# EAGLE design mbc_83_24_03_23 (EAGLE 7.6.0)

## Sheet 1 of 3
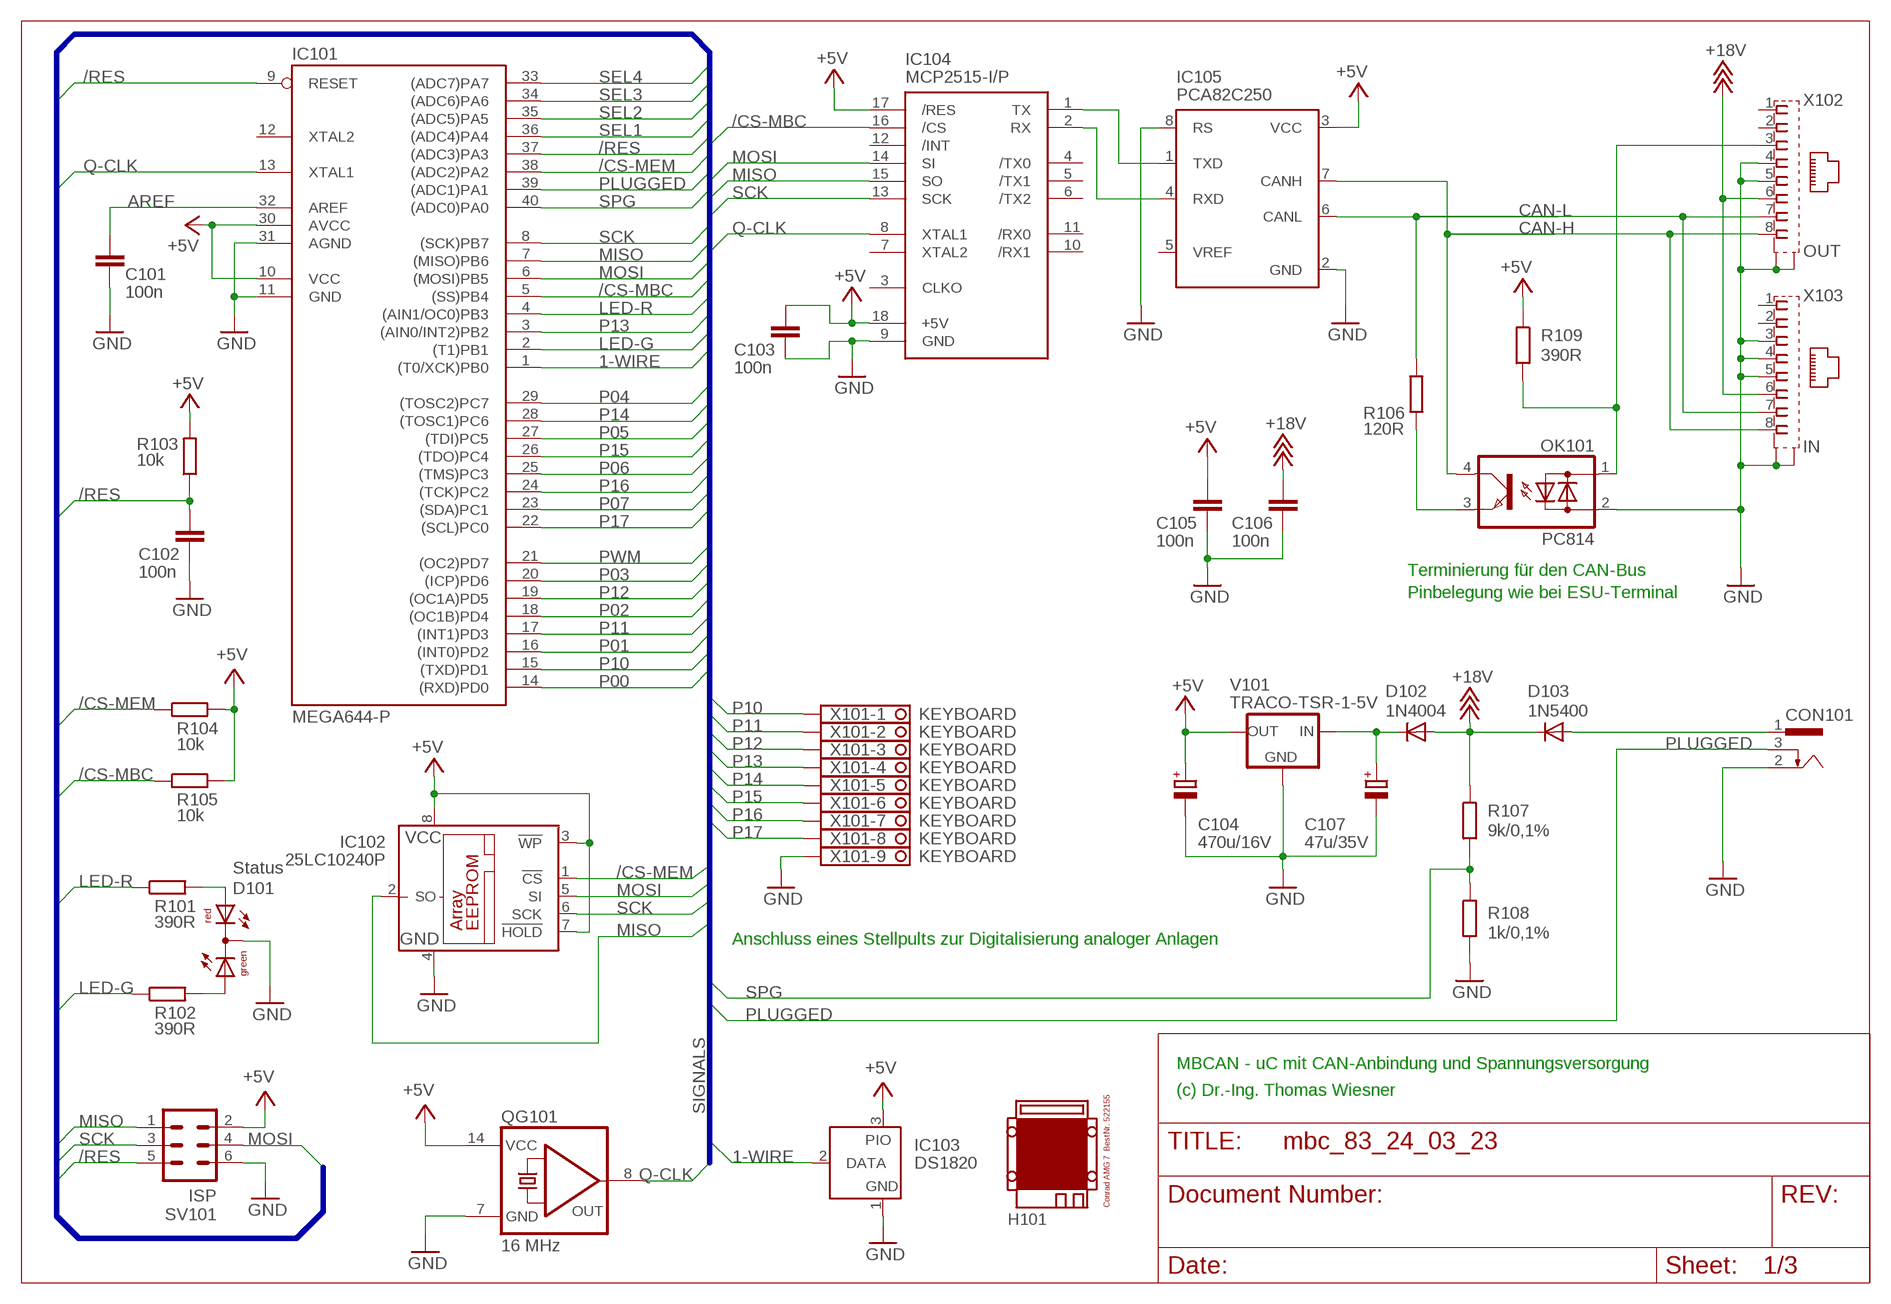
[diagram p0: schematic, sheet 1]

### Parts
C101  100n  C-EU025-025X050  [C025-025X050]
C102  100n  C-EU025-025X050  [C025-025X050]
C103  100n  C-EU025-025X050  [C025-025X050]
C104  470u/16V  CPOL-EUE3.5-8  [E3,5-8]
C105  100n  C-EU025-025X050  [C025-025X050]
C106  100n  C-EU025-025X050  [C025-025X050]
C107  47u/35V  CPOL-EUE2.5-7  [E2,5-7]
CON101  POWER-JACK  [POWER-JACK]
D101  Status  DUOLED5MM  [DUOLED5MM]
D102  1N4004  [DO41-10]
D103  1N5400  [DO201-15]
H101  MODULGEHÄUSE-AMG-7  [MODULGEHÄUSE-AMG-7]
IC101  MEGA644-P  MEGA323-P  [DIL40]
IC102  25LC10240P  25LC040P  [DIL8]
IC103  DS1820  DS2405  [TO92-]
IC104  MCP2515-I/P  MCP2510-I/P  [DIL18]
IC105  PCA82C250  [DIL08]
OK101  PC814  [DIL04]
QG101  16 MHz  QG5860  [DIL14S]
R101  390R  R-EU_0207/10  [0207/10]
R102  390R  R-EU_0207/10  [0207/10]
R103  10k  R-EU_0207/10  [0207/10]
R104  10k  R-EU_0207/10  [0207/10]
R105  10k  R-EU_0207/10  [0207/10]
R106  120R  R-EU_0207/10  [0207/10]
R107  9k/0,1%  R-EU_0207/10  [0207/10]
R108  1k/0,1%  R-EU_0207/10  [0207/10]
R109  390R  R-EU_0207/10  [0207/10]
SV101  ISP  ML6  [ML6]
V101  TRACO-TSR-1-5V  [TRACO-TSR-1]
X101  KEYBOARD  1751316  [1751316]
X102  OUT  0446200002  [0446200002]
X103  IN  0446200002  [0446200002]

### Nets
1-WIRE: IC101.1((T0/XCK)PB0) IC103.2(DATA)
+5V: C103.1 C104.+ C105.1 IC101.10(VCC) IC101.30(AVCC) IC102.3(!WP) IC102.7(!HOLD) IC102.8(VCC) IC103.3(PIO) IC104.17(/RES) IC104.18(+5V) IC105.3(VCC) QG101.14(VCC) R103.2 R104.2 R105.2 R109.1 SV101.2 V101.OUT ; also sheet 2
+18V: C106.1 D102.A D103.C R107.1 X102.6 X103.6 ; also sheet 2,3
/CS-MBC: IC101.5((SS)PB4) IC104.16(/CS) R105.1
/CS-MEM: IC101.38((ADC2)PA2) IC102.1(!CS) R104.1
/RES: C102.1 IC101.9(RESET) IC101.37((ADC3)PA3) R103.1 SV101.5
AREF: C101.1 IC101.32(AREF)
CAN-H: IC105.7(CANH) OK101.4(C) X102.8 X103.8
CAN-L: IC105.6(CANL) R106.2 X102.7 X103.7
GND: C101.2 C102.2 C103.2 C104.- C105.2 C106.2 C107.- CON101.2 D101.K(C) IC101.11(GND) IC101.31(AGND) IC102.4(GND) IC103.1(GND) IC104.9(GND) IC105.2(GND) IC105.8(RS) OK101.2(AC2) QG101.7(GND) R108.2 SV101.6 V101.GND X101.9 X102.4 X102.5 X102.S@1(S1) X102.S@2(S2) X103.3 X103.4 X103.5 X103.S@1(S1) X103.S@2(S2) ; also sheet 2,3
LED-G: IC101.2((T1)PB1) R102.1
LED-R: IC101.4((AIN1/OC0)PB3) R101.1
MISO: IC101.7((MISO)PB6) IC102.2(SO) IC104.15(SO) SV101.1
MOSI: IC101.6((MOSI)PB5) IC102.5(SI) IC104.14(SI) SV101.4
N$1: IC104.1(TX) IC105.1(TXD)
N$2: IC104.2(RX) IC105.4(RXD)
N$3: OK101.3(E) R106.1
N$5: OK101.1(AC1) R109.2 X102.3
N$6: C107.+ D102.C V101.IN
N$9: D101.AR R101.2
N$13: D101.AG R102.2
P00: IC101.14((RXD)PD0) ; also sheet 2
P01: IC101.16((INT0)PD2) ; also sheet 2
P02: IC101.18((OC1B)PD4) ; also sheet 2
P03: IC101.20((ICP)PD6) ; also sheet 2
P04: IC101.29((TOSC2)PC7) ; also sheet 2
P05: IC101.27((TDI)PC5) ; also sheet 2
P06: IC101.25((TMS)PC3) ; also sheet 2
P07: IC101.23((SDA)PC1) ; also sheet 2
P10: IC101.15((TXD)PD1) X101.1
P11: IC101.17((INT1)PD3) X101.2
P12: IC101.19((OC1A)PD5) X101.3
P13: IC101.3((AIN0/INT2)PB2) X101.4
P14: IC101.28((TOSC1)PC6) X101.5
P15: IC101.26((TDO)PC4) X101.6
P16: IC101.24((TCK)PC2) X101.7
P17: IC101.22((SCL)PC0) X101.8
PLUGGED: CON101.3 IC101.39((ADC1)PA1)
PWM: IC101.21((OC2)PD7) ; also sheet 3
Q-CLK: IC101.13(XTAL1) IC104.8(XTAL1) QG101.8(OUT)
SCK: IC101.8((SCK)PB7) IC102.6(SCK) IC104.13(SCK) SV101.3
SEL1: IC101.36((ADC4)PA4) ; also sheet 2
SEL2: IC101.35((ADC5)PA5) ; also sheet 2
SEL3: IC101.34((ADC6)PA6) ; also sheet 2
SEL4: IC101.33((ADC7)PA7) ; also sheet 2
SPG: IC101.40((ADC0)PA0) R107.2 R108.1
V-NETZTEIL1: CON101.1 D103.A
Unconnected: IC101.12(XTAL2) IC104.3(CLKO) IC104.4(/TX0) IC104.5(/TX1) IC104.6(/TX2) IC104.7(XTAL2) IC104.10(/RX1) IC104.11(/RX0) IC104.12(/INT) IC105.5(VREF) X102.1 X102.2 X103.1 X103.2

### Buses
SIGNALS

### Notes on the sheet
- Terminierung für den CAN-Bus
- Pinbelegung wie bei ESU-Terminal
- Anschluss eines Stellpults zur Digitalisierung analoger Anlagen
- MBCAN - uC mit CAN-Anbindung und Spannungsversorgung
- (c) Dr.-Ing. Thomas Wiesner

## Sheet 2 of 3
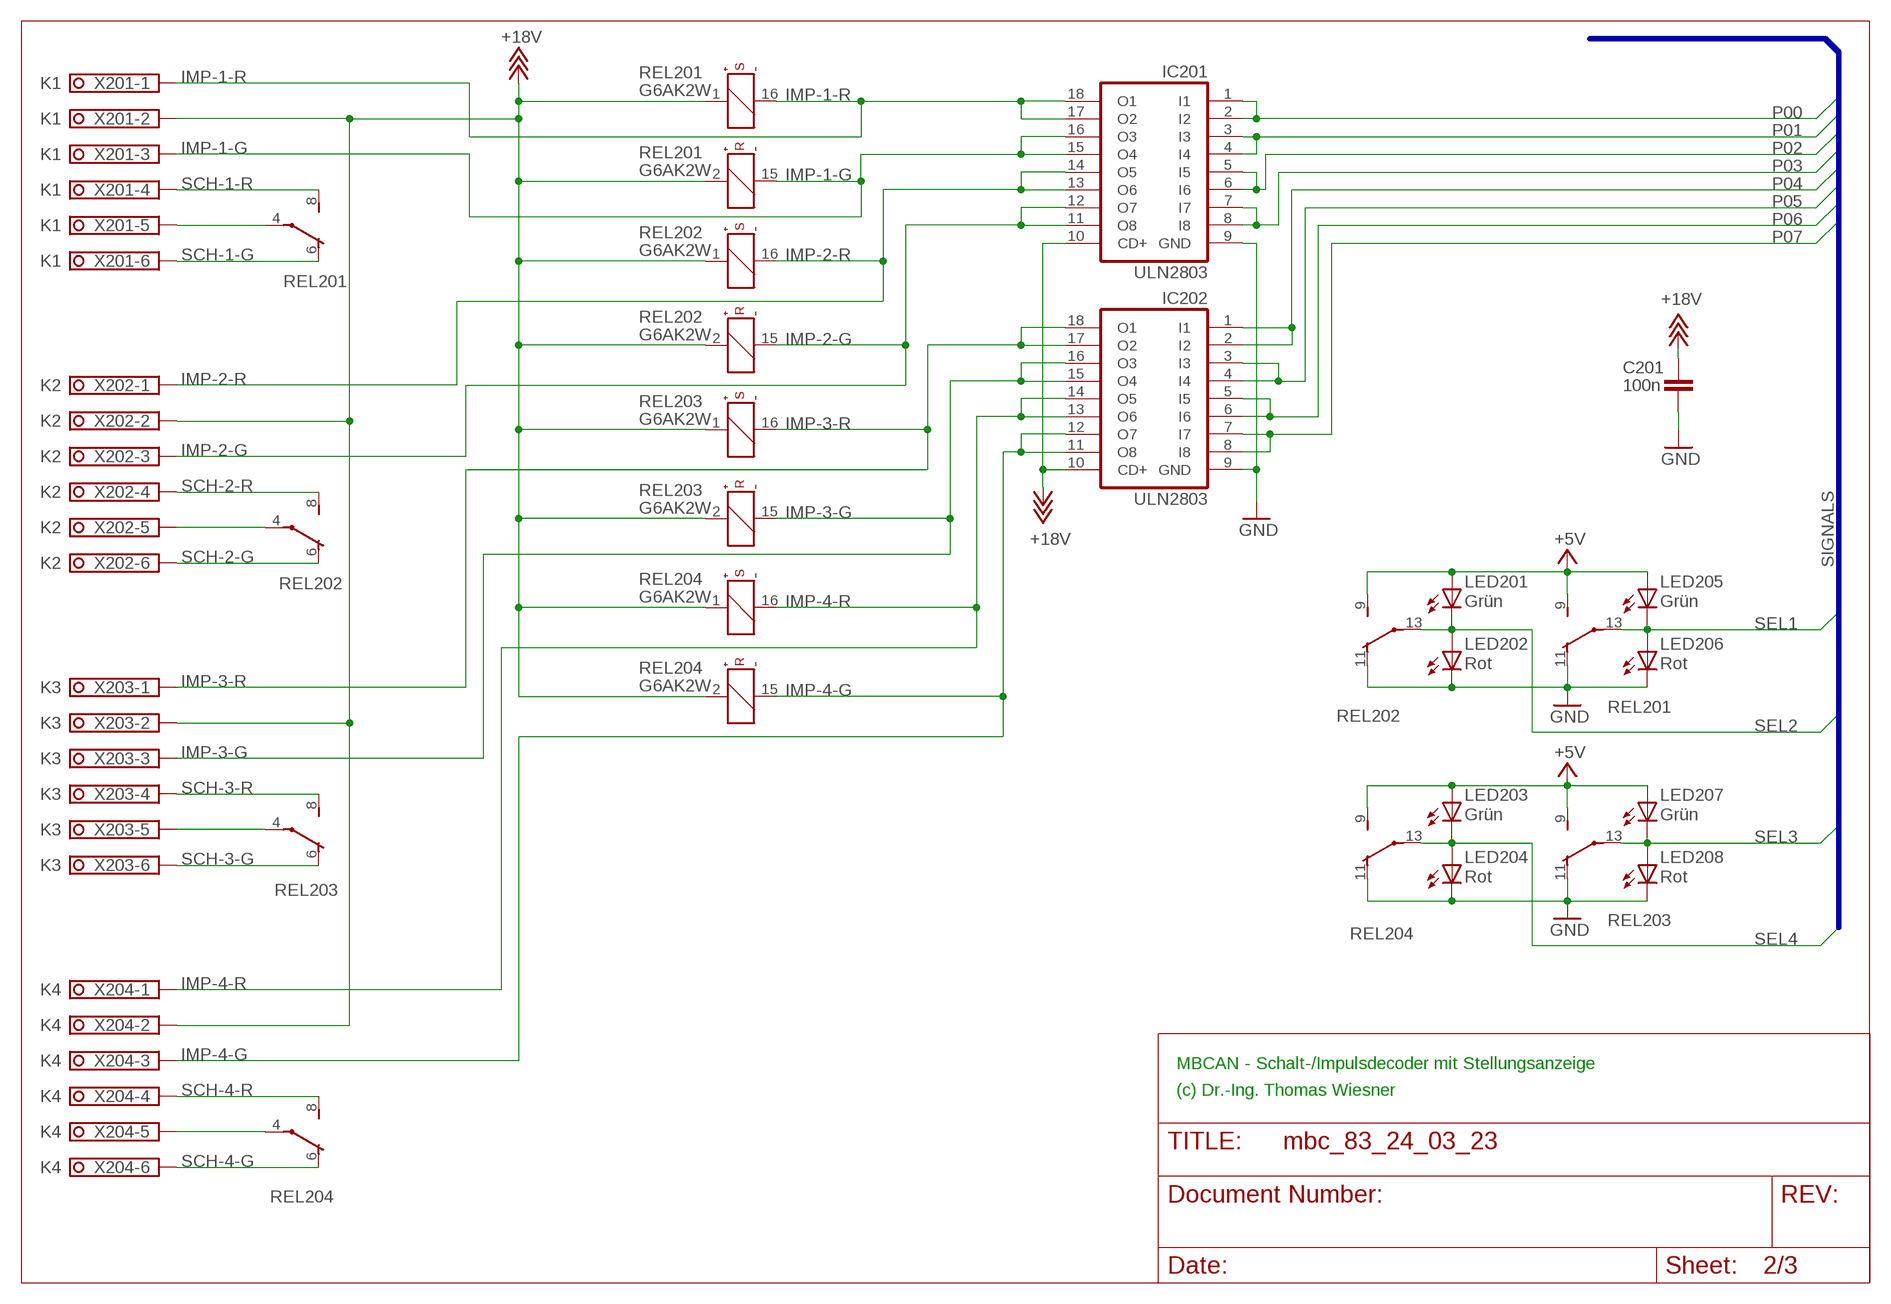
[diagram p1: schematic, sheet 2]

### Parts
C201  100n  C-EU025-025X050  [C025-025X050]
IC201  ULN2803  ULN2803A  [DIL18]
IC202  ULN2803  ULN2803A  [DIL18]
LED201  Grün  LED3MM  [LED3MM]
LED202  Rot  LED3MM  [LED3MM]
LED203  Grün  LED3MM  [LED3MM]
LED204  Rot  LED3MM  [LED3MM]
LED205  Grün  LED3MM  [LED3MM]
LED206  Rot  LED3MM  [LED3MM]
LED207  Grün  LED3MM  [LED3MM]
LED208  Rot  LED3MM  [LED3MM]
REL201  G6AK2W  [REL-BIPOLAR]
REL202  G6AK2W  [REL-BIPOLAR]
REL203  G6AK2W  [REL-BIPOLAR]
REL204  G6AK2W  [REL-BIPOLAR]
X201  K1  1751280  [1751280]
X202  K2  1751280  [1751280]
X203  K3  1751280  [1751280]
X204  K4  1751280  [1751280]

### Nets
+5V: LED201.A LED203.A LED205.A LED207.A REL201.9(S) REL202.9(S) REL203.9(S) REL204.9(S) ; also sheet 1
+18V: C201.1 IC201.10(CD+) IC202.10(CD+) REL201.1(+) REL201.2(+) REL202.1(+) REL202.2(+) REL203.1(+) REL203.2(+) REL204.1(+) REL204.2(+) X201.2 X202.2 X203.2 X204.2 ; also sheet 1,3
GND: C201.2 IC201.9(GND) IC202.9(GND) LED202.K(C) LED204.K(C) LED206.K(C) LED208.K(C) REL201.11(O) REL202.11(O) REL203.11(O) REL204.11(O) ; also sheet 1,3
IMP-1-G: IC201.15(O4) IC201.16(O3) REL201.15(-) X201.3 ; also sheet 3
IMP-1-R: IC201.17(O2) IC201.18(O1) REL201.16(-) X201.1 ; also sheet 3
IMP-2-G: IC201.11(O8) IC201.12(O7) REL202.15(-) X202.3 ; also sheet 3
IMP-2-R: IC201.13(O6) IC201.14(O5) REL202.16(-) X202.1 ; also sheet 3
IMP-3-G: IC202.15(O4) IC202.16(O3) REL203.15(-) X203.3 ; also sheet 3
IMP-3-R: IC202.17(O2) IC202.18(O1) REL203.16(-) X203.1 ; also sheet 3
IMP-4-G: IC202.11(O8) IC202.12(O7) REL204.15(-) X204.3 ; also sheet 3
IMP-4-R: IC202.13(O6) IC202.14(O5) REL204.16(-) X204.1 ; also sheet 3
N$12: REL202.4(P) X202.5
N$14: REL201.4(P) X201.5
N$15: REL203.4(P) X203.5
N$16: REL204.4(P) X204.5
P00: IC201.1(I1) IC201.2(I2) ; also sheet 1
P01: IC201.3(I3) IC201.4(I4) ; also sheet 1
P02: IC201.5(I5) IC201.6(I6) ; also sheet 1
P03: IC201.7(I7) IC201.8(I8) ; also sheet 1
P04: IC202.1(I1) IC202.2(I2) ; also sheet 1
P05: IC202.3(I3) IC202.4(I4) ; also sheet 1
P06: IC202.5(I5) IC202.6(I6) ; also sheet 1
P07: IC202.7(I7) IC202.8(I8) ; also sheet 1
SCH-1-G: REL201.6(O) X201.6 ; also sheet 3
SCH-1-R: REL201.8(S) X201.4
SCH-2-G: REL202.6(O) X202.6 ; also sheet 3
SCH-2-R: REL202.8(S) X202.4
SCH-3-G: REL203.6(O) X203.6 ; also sheet 3
SCH-3-R: REL203.8(S) X203.4
SCH-4-G: REL204.6(O) X204.6 ; also sheet 3
SCH-4-R: REL204.8(S) X204.4
SEL1: LED205.K(C) LED206.A REL201.13(P) ; also sheet 1
SEL2: LED201.K(C) LED202.A REL202.13(P) ; also sheet 1
SEL3: LED207.K(C) LED208.A REL203.13(P) ; also sheet 1
SEL4: LED203.K(C) LED204.A REL204.13(P) ; also sheet 1

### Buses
SIGNALS

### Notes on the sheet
- MBCAN - Schalt-/Impulsdecoder mit Stellungsanzeige
- (c) Dr.-Ing. Thomas Wiesner

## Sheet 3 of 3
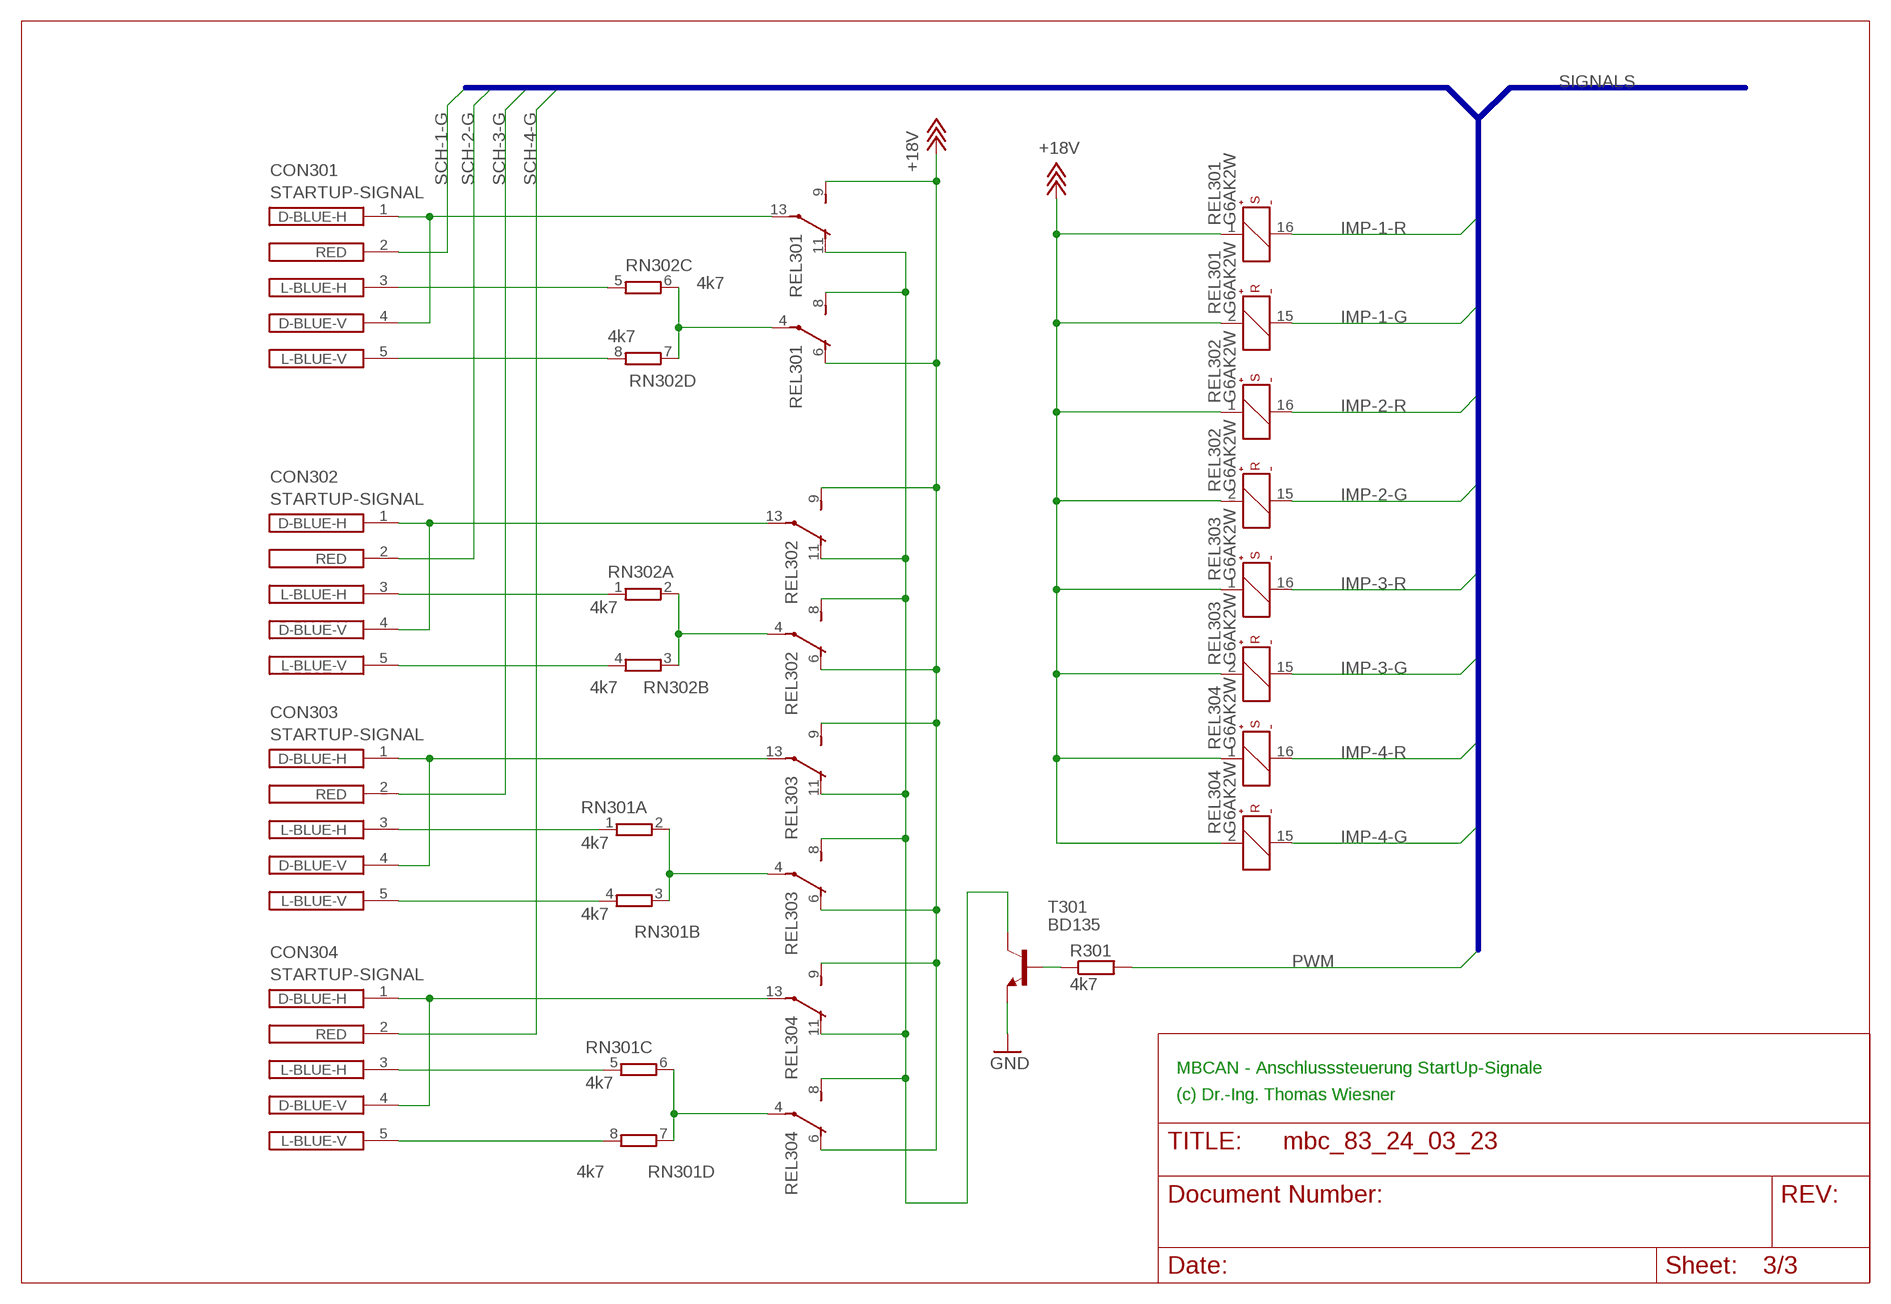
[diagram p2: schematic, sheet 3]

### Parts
CON301  STARTUP-SIGNAL  [SIGNAL-MAIN]
CON302  STARTUP-SIGNAL  [SIGNAL-MAIN]
CON303  STARTUP-SIGNAL  [SIGNAL-MAIN]
CON304  STARTUP-SIGNAL  [SIGNAL-MAIN]
R301  4k7  R-EU_0207/10  [0207/10]
REL301  G6AK2W  [REL-BIPOLAR]
REL302  G6AK2W  [REL-BIPOLAR]
REL303  G6AK2W  [REL-BIPOLAR]
REL304  G6AK2W  [REL-BIPOLAR]
RN301  4k7  E4R  [SIL8]
RN302  4k7  E4R  [SIL8]
T301  BD135  -NPN-TO126V  [TO126V]

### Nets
+18V: REL301.1(+) REL301.2(+) REL301.6(O) REL301.9(S) REL302.1(+) REL302.2(+) REL302.6(O) REL302.9(S) REL303.1(+) REL303.2(+) REL303.6(O) REL303.9(S) REL304.1(+) REL304.2(+) REL304.6(O) REL304.9(S) ; also sheet 1,2
GND: T301.1(E) ; also sheet 1,2
IMP-1-G: REL301.15(-) ; also sheet 2
IMP-1-R: REL301.16(-) ; also sheet 2
IMP-2-G: REL302.15(-) ; also sheet 2
IMP-2-R: REL302.16(-) ; also sheet 2
IMP-3-G: REL303.15(-) ; also sheet 2
IMP-3-R: REL303.16(-) ; also sheet 2
IMP-4-G: REL304.15(-) ; also sheet 2
IMP-4-R: REL304.16(-) ; also sheet 2
N$4: CON302.5(L-BLUE-V) RN302.4
N$7: CON301.1(D-BLUE-H) CON301.4(D-BLUE-V) REL301.13(P)
N$8: CON301.5(L-BLUE-V) RN302.8
N$10: CON303.5(L-BLUE-V) RN301.4
N$11: CON304.5(L-BLUE-V) RN301.8
N$17: R301.1 T301.3(B)
N$18: REL301.8(S) REL301.11(O) REL302.8(S) REL302.11(O) REL303.8(S) REL303.11(O) REL304.8(S) REL304.11(O) T301.2(C)
N$19: CON302.1(D-BLUE-H) CON302.4(D-BLUE-V) REL302.13(P)
N$20: CON302.3(L-BLUE-H) RN302.1
N$21: CON304.1(D-BLUE-H) CON304.4(D-BLUE-V) REL304.13(P)
N$23: CON304.3(L-BLUE-H) RN301.5
N$24: CON303.1(D-BLUE-H) CON303.4(D-BLUE-V) REL303.13(P)
N$26: CON301.3(L-BLUE-H) RN302.5
N$27: CON303.3(L-BLUE-H) RN301.1
N$29: REL301.4(P) RN302.6 RN302.7
N$30: REL302.4(P) RN302.2 RN302.3
N$31: REL303.4(P) RN301.2 RN301.3
N$32: REL304.4(P) RN301.6 RN301.7
PWM: R301.2 ; also sheet 1
SCH-1-G: CON301.2(RED) ; also sheet 2
SCH-2-G: CON302.2(RED) ; also sheet 2
SCH-3-G: CON303.2(RED) ; also sheet 2
SCH-4-G: CON304.2(RED) ; also sheet 2

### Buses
SIGNALS

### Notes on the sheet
- MBCAN - Anschlusssteuerung StartUp-Signale
- (c) Dr.-Ing. Thomas Wiesner

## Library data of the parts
C101-C103 C105 C106 C201 = rcl:C-EU: CAPACITOR, European symbol
C104 C107 = rcl:CPOL-EU: POLARIZED CAPACITOR, European symbol
CON101 = mbc:POWER-JACK: Power-Stecker für 2,5 mm Hohlbuchse
CON301-CON304 = mbc:STARTUP-SIGNAL: Connector für StartUp-Signale
D101 = led:DUOLED5MM: DUO LED 2 colors, 5 mm, round
D102 = diode:1N4004: DIODE
D103 = diode:1N5400: DIODE
H101 = mbc:MODULGEHÄUSE-AMG-7: Gehäuse
IC101 = atmel:MEGA323-P: MICROCONTROLLER 32 Kbytes FLASH 2 Kbytes SRAM 1 Kbytes EEPROM USART 8-channel 10 bit ADC Source: avr.lbr; OC_FARNELL: unknown; OC_NEWARK: unknown
IC102 = microchip:25*: Serial EEPROM 4K/ 8K , SPI bus; MF: MICROCHIP; MPN: 25LC040/P; OC_FARNELL: 9758100; OC_NEWARK: 96K4091
IC103 = maxim:DS2405: Addressable Switch DALLAS Semiconductor; MF: DALLAS SEMICONDUCTOR; MPN: DS2405; OC_FARNELL: 1188025; OC_NEWARK: 06F4645
IC104 = mbc:MCP2510: BASIC-CAN 2.0a Controller Stand-alone CAN controller von Microchip
IC105 = micro-philips:PCA82C250: CAN CONTROLLER INTERFACE; OC_FARNELL: 3692358; OC_NEWARK: unknown
IC201 IC202 = uln-udn:ULN2803A: DRIVER ARRAY
LED201-LED208 = led:LED: LED
OK101 = optocoupler:PC814: SHARP OPTO COUPLER; OC_FARNELL: 9707662; OC_NEWARK: unknown
QG101 = crystal:QG5860: CRYSTAL RESONATOR; OC_FARNELL: unknown; OC_NEWARK: unknown
R101-R109 R301 = resistor:R-EU_: RESISTOR, European symbol
REL201-REL204 REL301-REL304 = mbc:G6AK2W: Bipolares Relais 2xUM 12V
RN301 RN302 = resistor-sil:E4R: SIL RESISTOR; OC_FARNELL: unknown; OC_NEWARK: unknown
SV101 = con-ml:ML6: HARTING; OC_FARNELL: unknown; OC_NEWARK: unknown
T301 = transistor:*-NPN-: NPN Transistror BF959 corrected 2008.03.06
V101 = mbc:TRACO-TSR-1-5V: Spannungsregler Hersteller: TRACO Typ: TSR-1 5V: TSR 1-2450 Spg: 5V Strom: 1A Reichelt TSR 1-2450
X101 = con-phoenix-350:1751316: MKDS 1/ 9-3,5 Printklemme Nennstrom: 10 A Bemessungsspannung: 160 V Raster: 3,5 mm Polzahl: 9 Montageart: Löten Anschlussart: Schraubanschluss Anschlussrichtung vom Leiter zur Platine: 0° Source: http://eshop.phoenixcontact.com .. 1751316.pdf; OC_FARNELL: unknown; OC_NEWARK: unknown
X102 X103 = mbc:0446200002: RJ-45 INVERTED MODULAR JACK ASSEMBLY WITH RJ-11 KEEPOUT FEATURE Source: Data sheet MOLEX 0446200002 BUCHSE, RJ45, GESCHIRMT Source: Farnell; MF: MOLEX; MPN: 0446200002; OC_FARNELL: 9251910
X201-X204 = con-phoenix-350:1751280: MKDS 1/ 6-3,5 Printklemme Nennstrom: 10 A Bemessungsspannung: 160 V Raster: 3,5 mm Polzahl: 6 Montageart: Löten Anschlussart: Schraubanschluss Anschlussrichtung vom Leiter zur Platine: 0° Source: http://eshop.phoenixcontact.com .. 1751280.pdf; MPN: 1751280; OC_FARNELL: unknown; OC_NEWARK: 27R1765

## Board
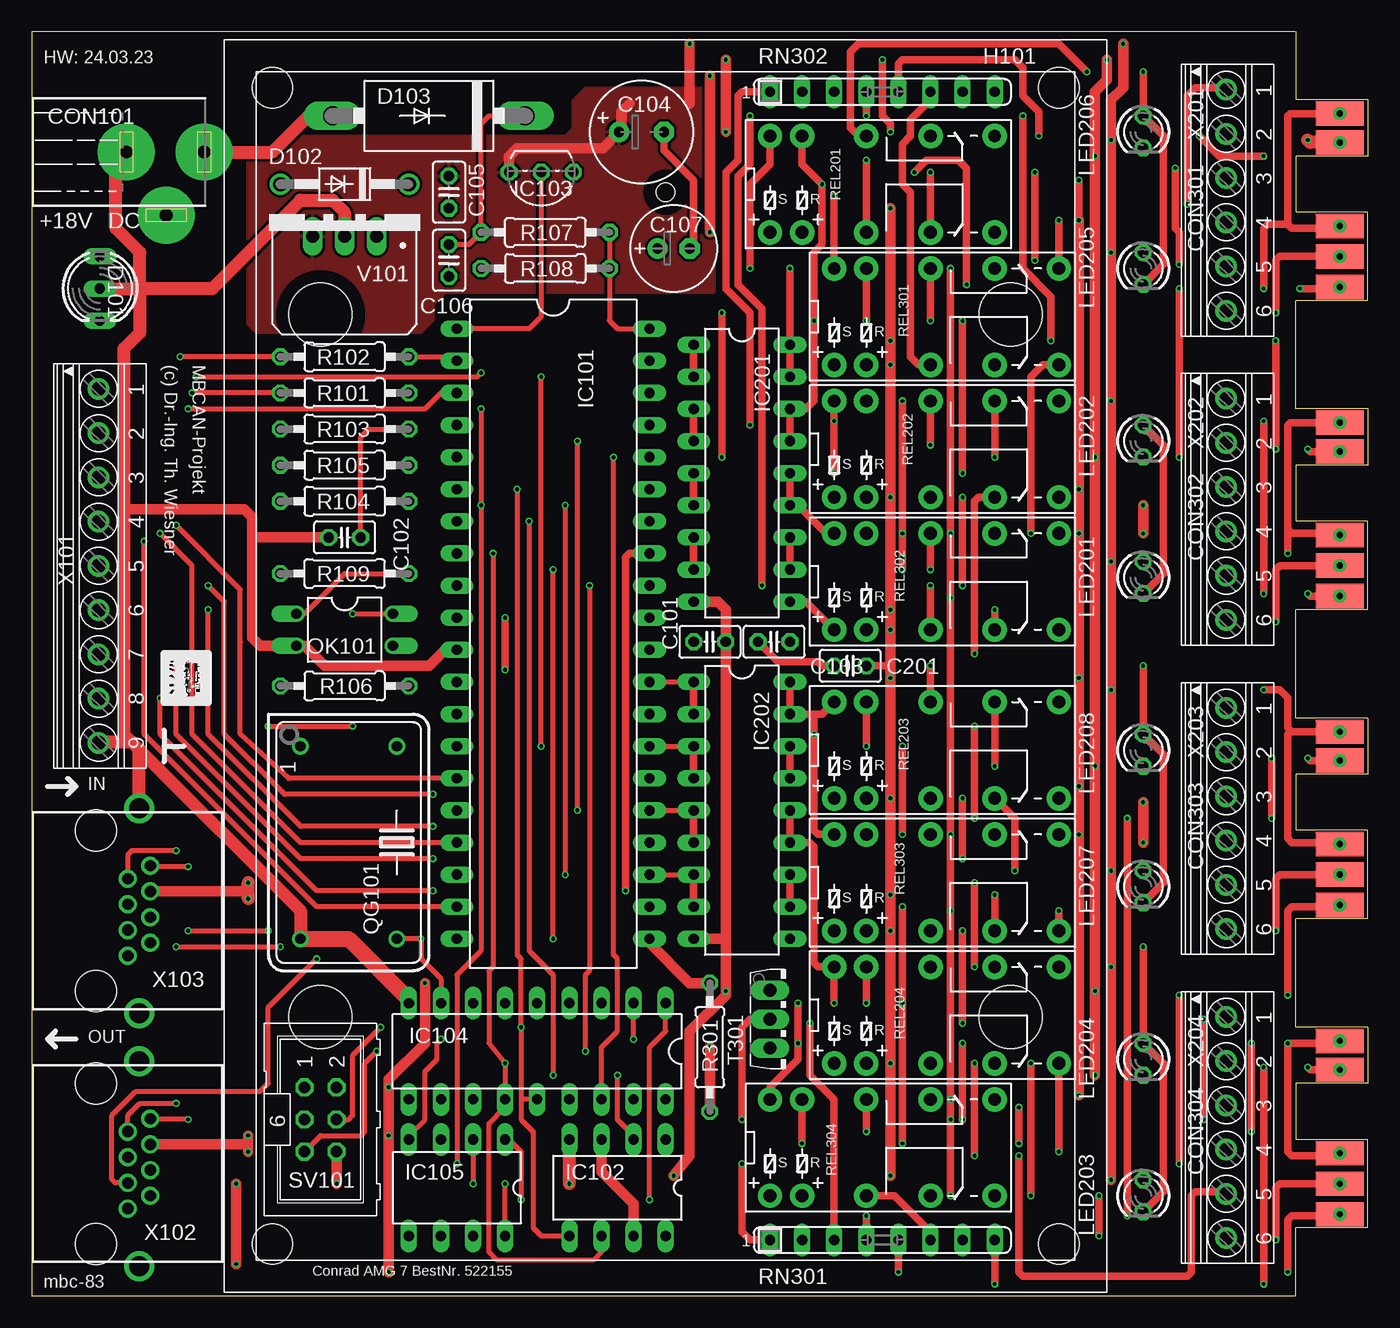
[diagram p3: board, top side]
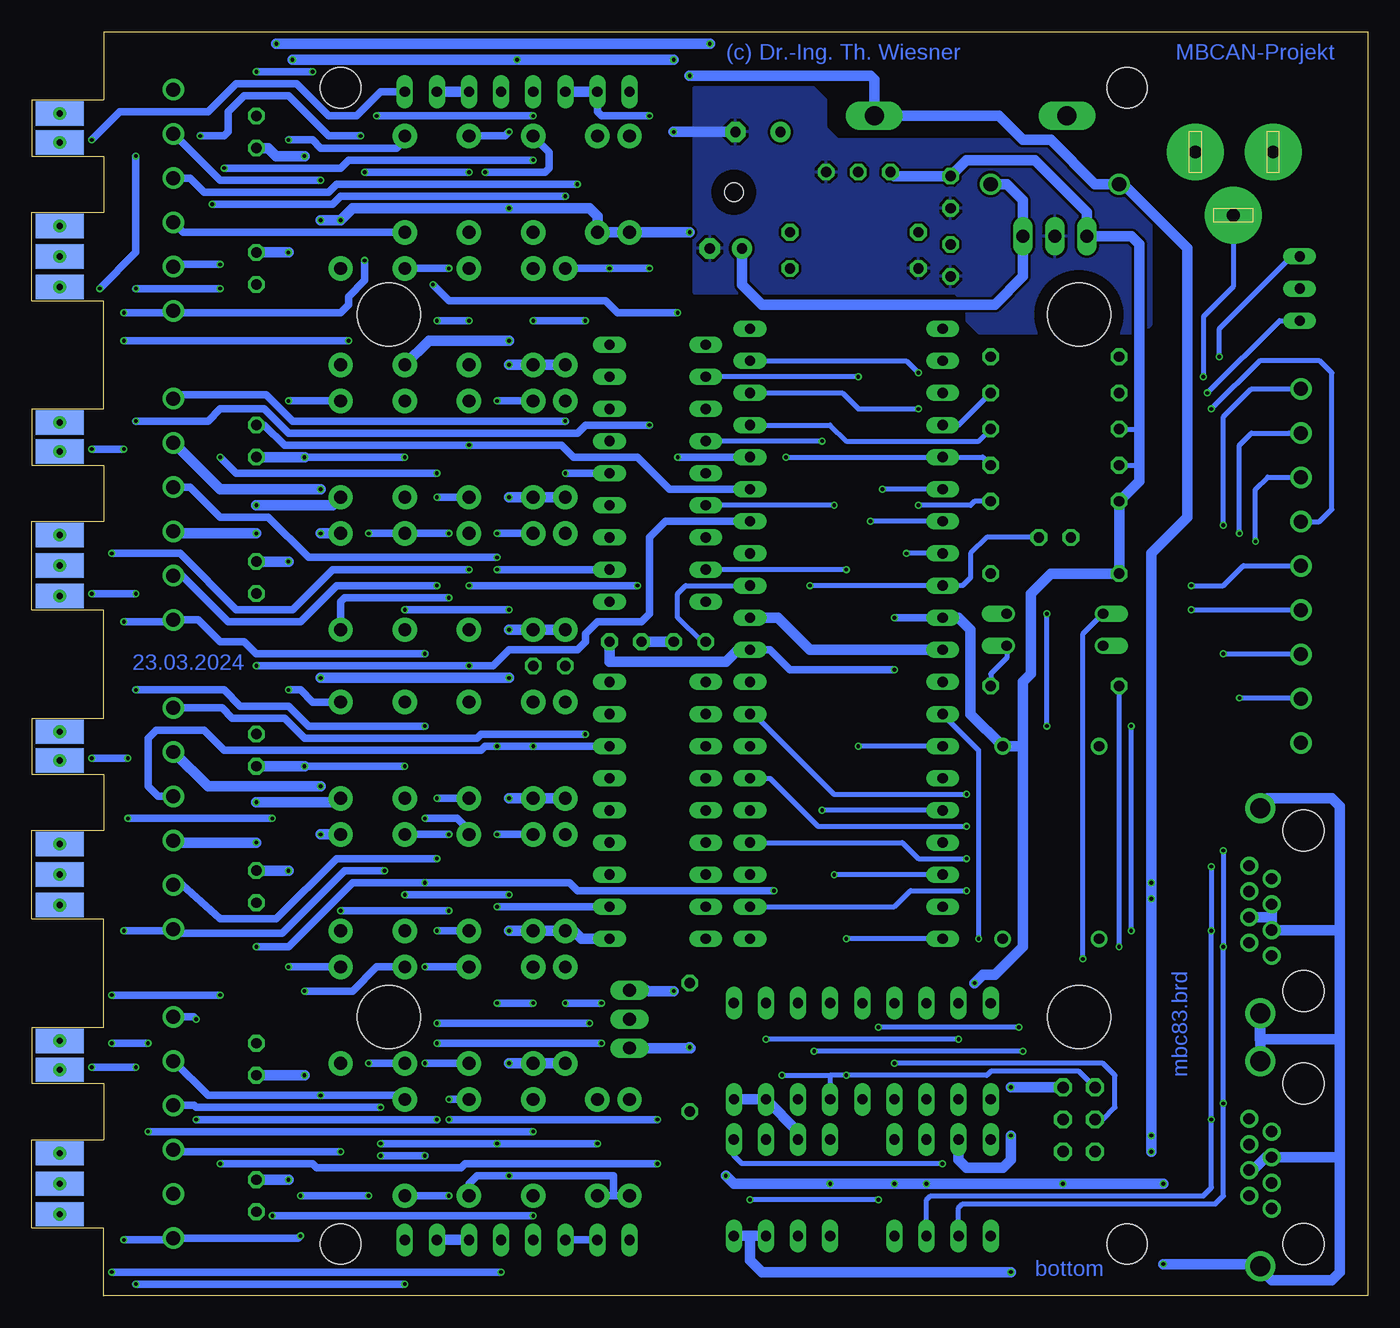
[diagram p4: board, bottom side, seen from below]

Size 105.73 x 100.01 mm. Coordinates in mm from the lower left corner, seen from the top.
Outline: 100,0.02 0,0.02 0,100.01 100,100.01
Outline: 100.01,100.01 100.01,94.61
Outline: 100.01,0 100.01,5.4
Outline: 100.01,21.27 100.01,29.84
Outline: 100.01,45.72 100.01,54.29
Outline: 100.01,70.17 100.01,78.74
Copper layers (1*16): Top 0.035mm / dielectric 1.5mm / Bottom 0.035mm
Design rules "default *": minimum track width 10mil, minimum drill 0.3mm, track to track 8mil, track to pad 8mil, pad to pad 8mil, via to via 8mil, smd to smd 8mil, copper to edge 40mil, drill to drill 8mil, minimum pad ring 10mil, minimum via ring 0.125mm, stop-mask expansion 4mil, vias tented up to drill 0mil, thermal gap 10mil

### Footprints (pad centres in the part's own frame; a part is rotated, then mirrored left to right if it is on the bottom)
C025-025X050 = drill 0.813 octagon: 1 -1.27,0; 2 1.27,0
E3,5-8 = drill 0.813 pad 1.6: + -1.778,0 | drill 0.813 pad 1.6 octagon: - 1.778,0
E2,5-7 = drill 0.813 pad 1.6: + -1.27,0 | drill 0.813 pad 1.6 octagon: - 1.27,0
POWER-JACK = drill 1 pad 4.5: 1 0,6.03; 2 0,-0.12; 3 5,3.03
SIGNAL-MAIN = smd 3.81 x 1.93: 1 -3.493,1.079; 2 -3.493,3.493; 3 -3.493,5.905; 4 -3.493,-7.811; 5 -3.493,-5.524 | smd 3.81 x 1.93 bottom: 6 -3.493,-5.524; 7 -3.493,-7.811; 8 -3.493,5.905; 9 -3.493,3.493; 10 -3.493,1.079 | drill 0.5 pad 0.813: P$7 -3.493,5.905; P$8 -3.493,3.493; P$9 -3.493,1.079; P$14 -3.493,-7.811; P$15 -3.493,-5.524
DUOLED5MM = drill 0.813 long: AG -2.54,0; AR 2.54,0; K 0,0
DO41-10 = drill 1.118: A 5.08,0; C -5.08,0
DO201-15 = drill 1.499 long: A 7.62,0; C -7.62,0
MODULGEHÄUSE-AMG-7 = hole 3.2: -45.72,-31.115; -45.72,31.115; 45.72,31.115; 45.72,-31.115 | hole 5: -27.781,-27.305; 27.781,-27.305; -27.781,27.305; 27.781,27.305 | hole 1.5: -37.465,0
DIL40 = drill 0.813 long: 1 -24.13,-7.62; 2 -21.59,-7.62; 3 -19.05,-7.62; 4 -16.51,-7.62; 5 -13.97,-7.62; 6 -11.43,-7.62; 7 -8.89,-7.62; 8 -6.35,-7.62; 9 -3.81,-7.62; 10 -1.27,-7.62; 11 1.27,-7.62; 12 3.81,-7.62; 13 6.35,-7.62; 14 8.89,-7.62; 15 11.43,-7.62; 16 13.97,-7.62; 17 16.51,-7.62; 18 19.05,-7.62; 19 21.59,-7.62; 20 24.13,-7.62; 21 24.13,7.62; 22 21.59,7.62; 23 19.05,7.62; 24 16.51,7.62; 25 13.97,7.62; 26 11.43,7.62; 27 8.89,7.62; 28 6.35,7.62; 29 3.81,7.62; 30 1.27,7.62; 31 -1.27,7.62; 32 -3.81,7.62; 33 -6.35,7.62; 34 -8.89,7.62; 35 -11.43,7.62; 36 -13.97,7.62; 37 -16.51,7.62; 38 -19.05,7.62; 39 -21.59,7.62; 40 -24.13,7.62
DIL8 = drill 0.813 long: 1 -3.81,-3.81; 2 -1.27,-3.81; 3 1.27,-3.81; 4 3.81,-3.81; 5 3.81,3.81; 6 1.27,3.81; 7 -1.27,3.81; 8 -3.81,3.81
TO92- = drill 0.813 octagon: 1 -2.54,0; 2 0,0; 3 2.54,0
DIL18 = drill 0.813 long: 1 -10.16,-3.81; 2 -7.62,-3.81; 3 -5.08,-3.81; 4 -2.54,-3.81 | drill 0.8 long: 5 0,-3.81; 6 2.54,-3.81; 7 5.08,-3.81; 8 7.62,-3.81; 9 10.16,-3.81; 10 10.16,3.81; 11 7.62,3.81; 12 5.08,3.81; 13 2.54,3.81; 14 0,3.81; 15 -2.54,3.81; 16 -5.08,3.81; 17 -7.62,3.81; 18 -10.16,3.81
DIL08 = drill 0.813 long: 1 -3.81,-3.81; 2 -1.27,-3.81; 3 1.27,-3.81; 4 3.81,-3.81; 5 3.81,3.81; 6 1.27,3.81; 7 -1.27,3.81; 8 -3.81,3.81
DIL18' = drill 0.813 long: 1 -10.16,-3.81; 2 -7.62,-3.81; 3 -5.08,-3.81; 4 -2.54,-3.81; 5 0,-3.81; 6 2.54,-3.81; 7 5.08,-3.81; 8 7.62,-3.81; 9 10.16,-3.81; 10 10.16,3.81; 11 7.62,3.81; 12 5.08,3.81; 13 2.54,3.81; 14 0,3.81; 15 -2.54,3.81; 16 -5.08,3.81; 17 -7.62,3.81; 18 -10.16,3.81
LED3MM = drill 0.813 octagon: A -1.27,0; K 1.27,0
DIL04 = drill 0.813 offset: 1 -1.27,-3.81; 2 1.27,-3.81; 3 1.27,3.81; 4 -1.27,3.81
DIL14S = drill 0.813: 1 -7.62,-3.81; 7 7.62,-3.81; 8 7.62,3.81; 14 -7.62,3.81
0207/10 = drill 0.813 octagon: 1 -5.08,0; 2 5.08,0
REL-BIPOLAR = drill 1.016 pad 1.93: 1 -8.89,-3.81; 2 -6.35,-3.81; 4 -1.27,-3.81; 6 3.81,-3.81; 8 8.89,-3.81; 9 8.89,3.81; 11 3.81,3.81; 13 -1.27,3.81; 15 -6.35,3.81; 16 -8.89,3.81
SIL8 = drill 0.813 long: 1 -8.89,0; 2 -6.35,0; 3 -3.81,0; 4 -1.27,0; 5 1.27,0; 6 3.81,0; 7 6.35,0; 8 8.89,0
ML6 = drill 0.914 octagon: 1 -2.54,-1.27; 2 -2.54,1.27; 3 0,-1.27; 4 0,1.27; 5 2.54,-1.27; 6 2.54,1.27
TO126V = drill 1.016 long: 1 -2.286,-1.27; 2 0,-1.27; 3 2.286,-1.27
TRACO-TSR-1 = drill 1.016 long: GND 0,2.54; IN -2.54,2.54; OUT 2.54,2.54
1751316 = drill 1.1 pad 1.7: 1 -13.973,-0.1; 2 -10.473,-0.1; 3 -6.973,-0.1; 4 -3.473,-0.1; 5 0.028,-0.1; 6 3.527,-0.1; 7 7.027,-0.1; 8 10.527,-0.1; 9 14.027,-0.1
0446200002 = drill 0.889 pad 1.422: 1 3.556,2.54; 2 2.54,4.318; 3 1.524,2.54; 4 0.508,4.318; 5 -0.508,2.54; 6 -1.524,4.318; 7 -2.54,2.54; 8 -3.556,4.318 | drill 1.575 pad 2.286: S@1 -8.103,3.429; S@2 8.103,3.429 | hole 3.251: 6.35,0; -6.35,0
1751280 = drill 1.1 pad 1.7: 1 -8.75,-0.1; 2 -5.25,-0.1; 3 -1.75,-0.1; 4 1.75,-0.1; 5 5.25,-0.1; 6 8.75,-0.1

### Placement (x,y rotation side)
C101  53.66,51.75 0 top
C102  24.77,60.01 180 top
C103  58.74,51.75 180 top
C104  48.26,92.08 0 top
C105  33.02,87.31 270 top
C106  33.02,81.92 270 top
C107  50.8,82.87 0 top
C201  64.77,49.85 180 top
CON101  7.62,90.49 270 top
CON301  100.01,85.72 180 top
CON302  100.01,61.28 180 top
CON303  100.01,36.83 180 top
CON304  100.01,12.38 180 top
D101  5.4,79.69 270 top
D102  24.77,87.95 180 top
D103  31.43,93.34 180 top
H101  50.16,49.85 270 top
IC101  41.27,52.39 270 top
IC102  46.35,8.57 180 top
IC103  40.32,88.9 180 top
IC104  40.01,19.37 180 top
IC105  33.66,8.57 180 top
IC201  ULN2803  [DIL18']  56.2,65.09 270 top
IC202  ULN2803  [DIL18']  56.2,38.42 270 top
LED201  87.95,56.83 270 top
LED202  87.95,67.63 270 top
LED203  87.95,7.94 270 top
LED204  87.95,18.73 270 top
LED205  87.95,81.28 270 top
LED206  87.95,92.08 270 top
LED207  87.95,32.38 270 top
LED208  87.95,43.18 270 top
OK101  24.77,52.7 270 top
QG101  25.08,35.88 270 top
R101  24.77,71.44 180 top
R102  24.77,74.3 180 top
R103  24.77,68.58 180 top
R104  24.77,62.87 180 top
R105  24.77,65.72 180 top
R106  24.77,48.26 180 top
R107  40.64,84.14 0 top
R108  40.64,81.28 180 top
R109  24.77,57.15 0 top
R301  53.66,19.68 90 top
REL201  67.31,87.95 0 top
REL202  72.39,66.99 0 top
REL203  72.39,43.18 0 top
REL204  72.39,22.23 0 top
REL301  72.39,77.47 0 top
REL302  72.39,56.52 0 top
REL303  72.39,32.7 0 top
REL304  67.31,11.75 0 top
RN301  67.31,4.45 0 top
RN302  67.31,95.25 0 top
SV101  22.86,13.97 270 top
T301  59.69,21.91 270 top
V101  24.77,86.36 180 top
X101  5.4,57.78 270 top
X102  5.08,10.48 270 top
X103  5.08,30.48 270 top
X201  94.61,86.68 270 top
X202  94.61,62.23 270 top
X203  94.61,37.78 270 top
X204  94.61,13.34 270 top

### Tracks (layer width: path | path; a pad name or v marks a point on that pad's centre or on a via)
1-WIRE
  Top 0.406: IC103.2 40.32,77.47 39.37,76.52 IC101.1
+5V  (via drill 0.3)
  Top 0.61: v37.47,49.53 v37.47,53.66
  Top 0.813: v31.11,24.77 31.11,20 28.26,17.14 v28.26,16.51 v28.26,12.7 v28.26,1.91 | 47.31,94.3 46.67,93.66 46.67,92.27 C104.+ 45.21,90.81 38.42,90.81 37.78,90.17 IC103.3 | IC102.3 45.09,9.84 47.62,7.3 IC102.7 | v85.41,9.21 v85.41,26.04 v85.41,33.66 v85.41,47.94 v85.41,58.1 v85.41,70.8 v85.41,82.55 v85.41,91.44 85.41,94.61 86.36,95.57 v86.36,99.06 | v52.07,99.06 52.07,94.3
  Bottom 0.406: R103.2 18.1,68.58 | R105.2 18.41,65.72 18.1,66.04
  Bottom 0.61: IC101.30 47.31,51.12 45.72,49.53 v37.47,49.53 | v37.47,53.66 IC101.10 | REL204.9 v85.41,26.04 | REL203.9 83.5,46.99 84.45,47.94 v85.41,47.94 | REL202.9 v85.41,70.8 | REL201.9 76.2,91.44 76.83,90.81 82.87,90.81 83.5,91.44 v85.41,91.44
  Bottom 0.813: v28.26,1.91 47.94,1.91 48.9,2.86 48.9,4.76 | IC101.10 32.38,53.66 31.43,52.7 31.43,46.04 QG101.14 27.3,43.5 | v28.26,12.7 28.26,10.79 28.89,10.16 31.75,10.16 32.38,10.79 IC105.3 | v31.11,24.77 30.48,25.4 29.53,25.4 27.3,27.62 27.3,43.5 | 48.9,4.76 IC102.7 | IC102.8 48.9,4.76 | IC104.18 IC104.17 45.09,13.02 IC102.3 | 27.3,43.5 27.3,48.58 26.67,49.21 26.67,55.56 25.08,57.15 R109.1 R104.2 18.1,64.45 18.1,66.04 18.1,68.58 18.1,83.19 18.73,83.82 V101.OUT 22.23,85.72 26.35,89.85 31.75,89.85 C105.1 37.47,88.58 IC103.3 | SV101.2 v28.26,16.51 | IC101.30 49.85,51.12 50.8,50.16 60.01,50.16 C103.1 | LED203.A v85.41,9.21 | v86.36,99.06 v52.07,99.06 | LED205.A v85.41,82.55 | LED201.A v85.41,58.1 | LED207.A v85.41,33.66
  pour Top: 17.14,76.83 17.14,91.76 42.23,91.76 42.86,92.39 42.86,94.61 43.81,95.57 53.98,95.57 53.98,79.38 32.7,79.38 31.75,78.42 31.75,77.15 30.8,76.2 17.78,76.2
+18V  (via drill 0.3)
  Top 0.406: C106.1 34.61,83.19 R107.1 35.56,92.71 36.2,93.34 D103.C
  Top 0.61: IC201.10 61.28,54.93 REL302.1 | REL301.9 v81.28,85.09 | v82.87,88.27 v82.87,85.09 | REL303.6 v76.2,31.75 | REL302.6 v76.2,54.29 | C201.1 67.63,49.85 67.94,49.53
  Top 0.813: v17.14,11.43 17.14,12.06 | 17.14,12.06 v17.14,12.7 | X102.6 17.08,12 17.14,12.06 | X103.6 16.9,32 | v67.94,86.04 v67.94,75.56 v67.94,73.66 v67.94,63.18 v67.94,54.29 v67.94,52.7 67.94,49.53 v67.94,48.9 v67.94,39.37 v67.94,31.75 v67.94,28.89 v67.94,18.41 v67.94,9.53 | v82.87,85.09 v82.87,63.82 v82.87,60.33 v82.87,48.9 v82.87,40.32 v82.87,36.51 v82.87,15.88 | v53.66,84.14 v53.66,96.52
  Top 1.016: 16.9,32 17.14,31.76 v17.14,31.43 v17.14,32.7
  Bottom 0.61: REL304.2 59.69,7.94 | 59.69,7.94 REL304.1 | 59.69,7.94 59.69,9.53 v67.94,9.53 70.48,9.53 71.12,8.89 REL304.6 | 94.47,18.59 91.76,15.88 v82.87,15.88 76.52,15.88 REL304.9 | 94.47,91.93 90.81,88.27 v82.87,88.27 | v76.2,31.75 v67.94,31.75 | v76.2,54.29 v67.94,54.29
  Bottom 0.813: v17.14,11.43 v17.14,12.7 v17.14,31.43 v17.14,32.7 17.14,58.74 14.29,61.59 14.29,82.87 19.37,87.95 D102.A 21.59,87.95 25.08,91.44 27.3,91.44 29.21,93.34 D103.C 39.05,96.2 39.37,96.52 v53.66,96.52 | v53.66,84.14 REL201.1 REL201.2 60.96,85.41 61.59,86.04 v67.94,86.04 80.33,86.04 v81.28,85.09 v82.87,85.09 | REL204.1 REL204.2 v67.94,18.41 | IC202.10 62.23,28.26 62.87,28.89 REL303.1 REL303.2 v67.94,28.89 | REL203.1 REL203.2 v67.94,39.37 | REL302.1 REL302.2 v67.94,52.7 | REL202.2 REL202.1 v67.94,63.18 | REL301.1 REL301.2 v67.94,73.66 | REL301.6 74.3,75.56 v67.94,75.56 | X204.2 94.47,18.59 | X203.2 94.47,43.03 91.76,40.32 v82.87,40.32 | X202.2 94.47,67.48 90.81,63.82 v82.87,63.82 | REL302.9 v82.87,60.33 | REL303.9 v82.87,36.51 | X201.2 94.47,91.93 | v82.87,48.9 v67.94,48.9
/CS-MBC  (via drill 0.3)
  Top 0.406: IC104.16 45.09,19.68 46.35,20.95 46.35,26.67 46.04,26.99 v46.04,66.36
  Bottom 0.406: R105.1 30.48,66.36 IC101.5 v46.04,66.36
/CS-MEM  (via drill 0.3)
  Top 0.406: v35.56,70.17 v35.56,62.55 35.56,27.3 33.66,25.4 v33.66,10.48
  Bottom 0.406: IC101.38 41.59,71.44 40.32,70.17 v35.56,70.17 | R104.1 31.11,62.87 31.43,62.55 v35.56,62.55 | v33.66,10.48 49.53,10.48 50.16,11.11 IC102.1
/RES  (via drill 0.3)
  Top 0.406: v44.13,56.2 44.13,25.72 43.81,25.4 v43.81,19.37 | C102.1 26.04,67.94 26.67,68.58 R103.1 | SV101.5 22.86,12.7 26.04,12.7 26.35,13.02 26.35,18.41 v27.3,19.37
  Bottom 0.406: IC101.37 42.55,68.9 41.27,67.63 30.8,67.63 R103.1 | v44.13,56.2 IC101.9 32.07,56.2 31.43,56.83 31.43,58.74 30.16,60.01 C102.1 | v27.3,19.37 v43.81,19.37
AREF
  Bottom 0.406: C101.1 52.7,51.75 54.61,53.66 54.61,55.56 53.98,56.2 IC101.32
CAN-H  (via drill 0.3)
  Top 0.406: X102.8 12.32,14.03 v12.38,13.97 | v12.38,33.97 9.46,33.97 X103.8 | v12.38,28.89 v18.73,28.89 | v18.73,45.09 v25.4,45.09 | v25.4,53.98 OK101.4
  Bottom 0.406: IC105.7 34.92,7.62 34.61,7.94 13.02,7.94 12.38,8.57 v12.38,13.97 v12.38,28.89 v12.38,33.97 | v18.73,28.89 v18.73,45.09 | v25.4,45.09 v25.4,53.98
CAN-L  (via drill 0.3)
  Top 0.406: X102.7 7.62,14.29 8.57,15.24 v11.43,15.24 | v11.43,35.24 7.94,35.24 7.62,34.92 X103.7 | v11.43,27.62 v19.68,27.62
  Bottom 0.406: IC105.6 32.38,6.99 32.07,7.3 12.06,7.3 11.43,7.94 v11.43,15.24 v11.43,27.62 v11.43,35.24 | v19.68,27.62 R106.2
GND  (via drill 0.3)
  Top 0.406: IC105.8 v37.47,8.89 | IC105.2 v34.92,8.89
  Top 0.61: C104.- 50.04,90.61 52.39,88.27 52.39,83.5 52.07,83.19 C107.- | 54.93,23.81 v54.93,24.13 | REL203.11 v76.2,41.91 | v76.2,66.36 REL202.11 | v67.94,92.08 67.94,92.71 67.31,93.34 v67.31,97.79 | C103.2 59.05,50.16 62.23,50.16 62.55,49.85 C201.2
  Top 0.813: 7.3,62.23 16.83,62.23 17.46,61.59 17.46,60.01 | 7.88,43.76 arc90 7.94,43.81 | IC202.9 54.93,28.26 | 54.93,28.26 v54.93,24.13 | 54.93,28.26 C101.2 54.93,54.29 54.29,54.93 IC201.9 | 17.46,60.01 17.46,52.07 18.1,51.44 OK101.2 21.59,51.44 23.18,49.85 31.43,49.85 32.7,51.12 IC101.11 | C102.2 17.46,60.01 | v50.8,9.53 52.07,11.11 52.07,20.95 54.93,23.81 | SV101.6 v24.13,8.89 | v16.19,2.54 v16.19,8.89 | v84.14,17.46 v84.14,24.13 v84.14,41.91 v84.14,66.36 v84.14,90.17 84.14,95.25 85.09,96.2 v85.09,97.79 | v54.93,97.79 v54.93,92.08
  Top 1.016: 8.57,79.69 14.29,79.69 21.27,86.68 23.81,86.68 24.77,85.72 V101.GND | D101.K 8.57,79.69 | 8.57,79.69 8.57,76.2 7.3,74.93 7.3,62.23 7.3,44.45 7.94,43.81 | v42.55,8.89 IC102.4 | 7.94,43.81 8.57,43.18 | 8.57,43.18 21.27,30.48 QG101.7 | 8.57,79.69 8.57,82.55 6.67,84.45 6.67,89.66 CON101.2 | 7.94,43.81 5.36,43.81 X101.9 | X103.S@1 8.51,43.12 8.57,43.18
  Top 1.27: IC104.9 29.84,23.5 25.08,28.26 QG101.7
  Bottom 0.61: 50.16,91.95 C104.- | X102.S@2 8.41,2.38 8.26,2.22 | REL204.11 78.42,26.04 80.33,24.13 v84.14,24.13 | v76.2,41.91 v84.14,41.91 | v84.14,66.36 v76.2,66.36 | REL201.11 68.26,91.76 v67.94,92.08
  Bottom 0.813: IC101.11 44.13,51.12 46.67,53.66 IC101.31 | v50.8,9.53 50.16,8.89 v42.55,8.89 v37.47,8.89 v34.92,8.89 v24.13,8.89 v16.19,8.89 | X102.S@2 8.67,2.54 v16.19,2.54 | 8.26,2.22 8.26,1.91 7.62,1.27 2.86,1.27 2.22,1.91 2.22,11.11 | 2.22,11.11 2.22,20.32 | 2.22,20.32 2.22,28.89 | 2.22,28.89 2.22,38.73 2.86,39.37 7.94,39.37 8.57,38.73 8.57,38.65 X103.S@1 | X102.S@1 X103.S@2 8.57,22.31 8.57,20.32 2.22,20.32 | 2.22,28.89 2.29,28.96 X103.3 7.62,30.16 | X103.5 7.62,30.16 | X103.4 7.81,29.97 7.62,30.16 | 2.22,11.11 2.35,10.99 X102.5 8.06,10.99 8.89,10.16 9.21,10.16 X102.4 | C103.2 C101.2 | 58.48,24.13 T301.1 57.09,24.19 56.83,24.13 v54.93,24.13 | LED204.K v84.14,17.46 | v85.09,97.79 v67.31,97.79 v54.93,97.79 | v54.93,92.08 C104.- | LED206.K 87,90.81 86.36,90.17 v84.14,90.17 | LED202.K v84.14,66.36 | LED208.K v84.14,41.91
  pour Bottom: 17.78,91.44 41.91,91.44 42.86,92.39 42.86,94.61 43.81,95.57 53.34,95.57 53.34,79.38 32.7,79.38 31.75,78.42 31.75,77.15 30.8,76.2 17.78,76.2 17.14,76.83 17.14,90.81
IMP-1-G  (via drill 0.3)
  Top 0.61: IC201.15 IC201.16 61.28,70.17 61.91,70.8 v61.91,77.15 61.91,82.55 62.55,83.19 v62.55,87.95 60.96,89.53 REL201.15 | v66.04,77.15 REL301.15
  Bottom 0.61: v61.91,77.15 v66.04,77.15 | X201.3 93.19,88.43 92.08,87.31 82.23,87.31 81.6,87.95 v62.55,87.95
IMP-1-R  (via drill 0.3)
  Top 0.61: IC201.17 IC201.18 v60.01,81.28 | REL201.16 58.42,89.53 56.83,87.95 v56.83,81.28 | REL301.16 v63.5,87 | v91.44,86.36 91.44,94.93 92.08,95.57 94.38,95.57 X201.1
  Bottom 0.61: REL301.16 v60.01,81.28 v56.83,81.28 | v63.5,87 81.28,87 81.92,86.36 v91.44,86.36
IMP-2-G  (via drill 0.3)
  Top 0.61: IC201.11 IC201.12 | v68.9,70.8 v68.9,60.33 v68.9,58.42 v68.9,57.47
  Bottom 0.61: REL202.15 v68.9,70.8 | v68.9,57.47 IC201.11 | REL302.15 v68.9,60.33 | X202.3 93.19,63.98 90.81,61.59 87,61.59 83.82,58.42 v68.9,58.42
IMP-2-R  (via drill 0.3)
  Top 0.61: IC201.14 IC201.13 60.64,62.55 62.87,60.33 REL302.16 | v63.5,65.09 v63.5,69.22 REL202.16
  Bottom 0.61: IC201.14 v63.5,65.09 | v63.5,69.22 85.09,69.22 87.17,71.3 94.2,71.3 X202.1
IMP-3-G  (via drill 0.3)
  Top 0.61: IC202.16 IC202.15 | v68.9,43.5 v68.9,36.51 | REL203.15 v66.04,43.5
  Bottom 0.61: IC202.16 v66.04,43.5 v68.9,43.5 69.85,43.5 70.17,43.18 90.49,43.18 92.08,44.77 95.89,44.77 96.52,44.13 96.52,40.32 95.73,39.53 X203.3 | v68.9,36.51 REL303.15
IMP-3-R  (via drill 0.3)
  Top 0.61: IC202.18 IC202.17 61.91,46.04 | 61.91,46.04 v61.91,44.45 61.91,36.83 62.23,36.51 REL303.16 | 61.91,46.04 62.55,46.04 REL203.16
  Bottom 0.61: X203.1 90.67,46.53 89.85,45.72 85.72,45.72 84.14,44.13 70.48,44.13 70.17,44.45 v61.91,44.45
IMP-4-G  (via drill 0.3)
  Top 0.61: IC202.11 IC202.12 | REL204.15 v66.04,23.18 | v68.9,30.8 v68.9,23.18 v68.9,12.06 | v78.11,14.92 v78.11,12.06 | v60.96,12.06 REL304.15
  Bottom 0.61: IC202.11 v68.9,30.8 | X204.3 92.87,15.09 92.71,14.92 v78.11,14.92 | v78.11,12.06 v68.9,12.06 v60.96,12.06 | v66.04,23.18 v68.9,23.18
IMP-4-R  (via drill 0.3)
  Top 0.61: IC202.14 IC202.13 61.59,35.88 61.91,35.56 61.91,26.35 62.23,26.04 REL204.16 v63.5,23.18 | v60.64,23.18 v60.64,20 60.64,18.73 58.42,16.51 REL304.16 | v92.71,21.91 v92.71,13.97 | v73.66,13.97 v73.66,20
  Bottom 0.61: v63.5,23.18 v60.64,23.18 | X204.1 92.89,22.09 v92.71,21.91 | v92.71,13.97 v73.66,13.97 | v73.66,20 v60.64,20
LED-G
  Top 0.406: R102.1 32.7,74.3 33.02,73.98 IC101.2
LED-R
  Bottom 0.406: IC101.4 32.38,68.9 R101.1
MISO  (via drill 0.3)
  Top 0.406: IC102.2 47.62,12.7 46.35,13.97 v46.35,17.46 | v39.37,61.28 39.37,27.3 41.27,25.4 v41.27,17.46
  Bottom 0.406: SV101.1 22.86,17.78 29.84,17.78 30.16,17.46 v41.27,17.46 42.55,17.46 | 42.55,17.46 IC104.15 | v46.35,17.46 42.55,17.46 | IC101.7 v39.37,61.28
MOSI  (via drill 0.3)
  Top 0.406: v38.42,63.82 38.42,26.99 38.73,26.67 v38.73,21.27 38.73,15.56 | SV101.4 25.08,13.97 25.4,14.29 25.4,19.05 v27.62,21.27 | 38.73,15.56 38.73,13.97 39.69,13.02 39.69,5.4 40.32,4.76 IC102.5 | IC104.14 38.73,15.56
  Bottom 0.406: IC101.6 v38.42,63.82 | v27.62,21.27 v38.73,21.27
N$1  (via drill 0.3)
  Top 0.406: IC105.1 37.78,12.38 38.73,11.43 v38.73,7.62 | v48.9,7.62 48.9,19.68 50.16,20.95 IC104.1
  Bottom 0.406: v38.73,7.62 v48.9,7.62
N$2  (via drill 0.3)
  Top 0.406: IC105.4 29.84,12.7 31.11,13.97 31.11,17.78 32.07,18.73 32.07,20 v32.38,20.32 | v47.62,20.32 IC104.2
  Bottom 0.406: v32.38,20.32 v47.62,20.32
N$3
  Bottom 0.406: OK101.3 28.57,50.48 29.84,49.21 R106.1
N$4  (via drill 0.3)
  Top 0.61: CON302.5 101.16,66.8 v100.97,66.99 | v98.42,66.99 v98.42,75.56 | v80.64,75.56 80.64,79.06 78.42,81.28 v78.42,93.34 | v66.04,93.34 RN302.4
  Bottom 0.61: v100.97,66.99 v98.42,66.99 | v98.42,75.56 v80.64,75.56 | v78.42,93.34 v66.04,93.34
N$5  (via drill 0.3)
  Top 0.406: OK101.1 21.59,53.98 24.77,57.15 R109.2 | X102.3 6.6,8.95 6.35,9.21 6.35,14.29 8.26,16.19 18.1,16.19 18.73,16.83 18.73,22.86 v22.54,26.67
  Bottom 0.406: v22.54,26.67 22.54,52.39 OK101.1
N$6
  Bottom 0.813: D102.C 28.57,87.95 27.3,86.68 V101.IN 27.3,80.64 29.53,78.42 47.94,78.42 49.53,80.01 C107.+
N$7  (via drill 0.3)
  Top 0.61: CON301.4 99.57,93.53 99.38,93.34 99.38,84.77 | 99.38,84.77 99.69,84.45 103.31,84.45 CON301.1 | REL301.13 v71.12,77.15 | v73.66,77.15 v73.66,65.09 | v90.81,66.36 v90.81,79.69 | v97.47,79.69 97.47,84.45 97.79,84.77 99.38,84.77
  Bottom 0.61: v71.12,77.15 v73.66,77.15 | v73.66,65.09 89.53,65.09 v90.81,66.36 | v90.81,79.69 v97.47,79.69
N$8  (via drill 0.3)
  Top 1.016: CON301.5 101.16,91.25 v100.97,91.44
  Bottom 0.61: RN302.8 78.11,95.25 80.01,93.34 82.23,93.34 84.77,95.89 89.53,95.89 91.76,93.66 98.74,93.66 v100.97,91.44
N$9  (via drill 0.3)
  Top 0.406: R101.2 v12.7,71.44
  Bottom 0.406: v12.7,71.44 6.99,77.15 D101.AR
N$10  (via drill 0.3)
  Top 0.61: CON303.5 101.16,42.35 v100.97,42.55 | RN301.4 v66.04,6.35 | v86.68,6.35 v86.68,37.78 | v98.11,37.78 v98.11,42.55
  Bottom 0.61: v66.04,6.35 v86.68,6.35 | v86.68,37.78 v98.11,37.78 | v98.11,42.55 v100.97,42.55
N$11  (via drill 0.3)
  Top 0.61: CON304.5 101.16,17.91 v100.97,18.1 | RN301.8 v76.2,0.95 | v97.47,0.95 v97.47,18.1
  Bottom 0.61: v76.2,0.95 v97.47,0.95 | v97.47,18.1 v100.97,18.1
N$12  (via drill 0.3)
  Top 0.61: v73.66,56.2 v73.66,63.18
  Bottom 0.61: X202.5 93.81,56.98 90.17,53.34 84.45,53.34 81.6,56.2 v73.66,56.2 | v73.66,63.18 REL202.4
N$13  (via drill 0.3)
  Top 0.406: R102.2 v11.75,74.3
  Bottom 0.406: v11.75,74.3 11.75,76.52 6.03,82.23 D101.AG
N$14  (via drill 0.3)
  Top 0.61: v90.81,81.6 90.81,84.14 90.49,84.45 v90.49,89.22 | v66.04,89.85 REL201.4
  Bottom 0.61: X201.5 94.47,81.43 94.3,81.6 v90.81,81.6 | v90.49,89.22 81.28,89.22 80.64,89.85 v66.04,89.85
N$15  (via drill 0.3)
  Top 0.61: v73.66,34.61 v73.66,39.37
  Bottom 0.61: X203.5 93.81,32.53 90.81,29.84 86.36,29.84 81.6,34.61 v73.66,34.61 | v73.66,39.37 REL203.4
N$16  (via drill 0.3)
  Top 0.61: v74.61,18.41 v74.61,11.11 | v78.11,11.11 78.11,1.91 78.42,1.59 91.44,1.59 91.76,1.91 91.76,7.94 92.08,8.26 94.34,8.26 X204.5
  Bottom 0.61: REL204.4 v74.61,18.41 | v74.61,11.11 v78.11,11.11
N$17  (via drill 0.3)
  Top 0.813: v53.66,19.68 R301.1
  Bottom 0.813: T301.3 53.59,19.62 v53.66,19.68
N$18  (via drill 0.3)
  Top 0.61: v72.71,81.28 v72.71,60.33 v72.71,55.24 v72.71,36.51 v72.71,30.48 v72.71,15.56 v72.71,13.97 v72.71,7.94 | T301.2 56.83,21.91 56.2,21.27 v56.2,13.97 | REL303.8 v81.28,30.48 | REL301.8 80.01,73.66 79.06,72.71 v79.06,60.33
  Bottom 0.61: REL304.11 v72.71,15.56 | v72.71,81.28 REL301.11 | v72.71,7.94 REL304.8 | v56.2,13.97 v72.71,13.97 | v81.28,30.48 v72.71,30.48 | REL303.11 v72.71,36.51 | REL302.8 81.28,54.93 80.96,55.24 v72.71,55.24 | v72.71,60.33 REL302.11 v79.06,60.33
N$19  (via drill 0.3)
  Top 0.61: CON302.4 99.57,69.09 99.38,68.9 99.38,60.64 | 99.38,60.64 99.69,60.33 103.38,60.33 CON302.1 | REL302.13 v71.12,57.47 | v99.38,58.74 99.38,60.64
  Bottom 0.61: v71.12,57.47 81.92,57.47 85.09,54.29 89.53,54.29 93.98,58.74 v99.38,58.74
N$20  (via drill 0.3)
  Top 0.61: CON302.3 101.16,55.37 v100.97,55.56 | v97.47,55.56 v97.47,69.22 | v56.83,68.9 56.83,77.79 54.93,79.69 54.93,88.9 55.88,89.85 55.88,94.93 56.2,95.25 RN302.1
  Bottom 0.61: v100.97,55.56 v97.47,55.56 | v97.47,69.22 91.76,69.22 90.81,70.17 87.31,70.17 85.41,68.26 62.55,68.26 61.91,68.9 v56.83,68.9
N$21  (via drill 0.3)
  Top 0.61: CON304.1 102.11,11.3 101.92,11.11 99.69,11.11 99.38,11.43 v99.38,20 103.31,20 CON304.4 | v96.52,20 v96.52,13.02 | v66.04,13.02 REL304.13
  Bottom 0.61: v99.38,20 v96.52,20 | v96.52,13.02 v66.04,13.02
N$23  (via drill 0.3)
  Top 0.61: v99.38,1.91 99.38,6.03 99.69,6.35 103.38,6.35 CON304.3 | v68.58,1.91 RN301.5
  Bottom 0.61: v99.38,1.91 v68.58,1.91
N$24  (via drill 0.3)
  Top 0.61: CON303.4 99.69,44.64 | 99.69,44.64 99.57,44.64 99.38,44.45 99.38,36.2 99.69,35.88 103.38,35.88 CON303.1 | v74.61,37.78 v74.61,45.09 | v97.47,47.94 98.74,47.94 99.38,47.31 99.38,44.96 99.69,44.64
  Bottom 0.61: REL303.13 71.12,36.83 72.07,37.78 v74.61,37.78 | v74.61,45.09 83.82,45.09 85.41,46.67 89.22,46.67 90.49,47.94 v97.47,47.94
N$26  (via drill 0.3)
  Top 0.61: RN302.5 68.58,97.47 68.9,97.79 77.79,97.79 78.42,97.16 78.42,94.93 79.69,93.66 v79.69,91.76 | v92.39,91.76 93.98,90.17 v97.47,90.17 | v100.33,79.69 103.38,79.69 CON301.3
  Bottom 0.61: v79.69,91.76 82.23,91.76 85.41,94.93 88.9,94.93 90.17,93.66 90.17,92.08 90.49,91.76 v92.39,91.76 | v97.47,90.17 97.47,82.55 v100.33,79.69
N$27  (via drill 0.3)
  Top 0.61: RN301.1 56.83,4.45 56.2,5.08 v56.2,10.48 | v90.81,10.48 v90.81,23.81 | v99.38,23.81 99.38,30.48 99.69,30.8 103.38,30.8 CON303.3
  Bottom 0.61: v56.2,10.48 71.44,10.48 71.75,10.16 83.19,10.16 83.5,10.48 v90.81,10.48 | v90.81,23.81 v99.38,23.81
N$29
  Top 0.61: RN302.6 71.12,94.61 69.53,93.03 69.53,91.76 68.9,91.12 68.9,87.95 69.53,87.31 69.53,74.3 70.17,73.66 REL301.4
  Bottom 0.813: RN302.7 RN302.6
N$30  (via drill 0.3)
  Top 0.61: REL302.4 v71.12,56.2 | v57.78,56.2 57.78,78.11 55.88,80.01 55.88,88.58 56.83,89.53 v56.83,93.34
  Bottom 0.61: v71.12,56.2 v57.78,56.2 | v56.83,93.34 60.64,93.34 60.96,93.66 RN302.2
  Bottom 0.813: RN302.2 RN302.3
N$31  (via drill 0.3)
  Top 0.61: RN301.3 63.5,15.56 61.59,17.46 v61.59,21.59 | v73.66,21.59 v73.66,28.89
  Bottom 0.61: RN301.2 RN301.3 | v61.59,21.59 v73.66,21.59 | v73.66,28.89 REL303.4
N$32
  Top 0.61: REL304.4 68.26,7.94 71.12,5.08 RN301.6
  Bottom 0.813: RN301.7 RN301.6
P00  (via drill 0.3)
  Top 0.406: v40.32,43.5 v40.32,72.71
  Top 0.61: IC201.2 IC201.1
  Bottom 0.406: IC101.14 v40.32,43.5 | v40.32,72.71 IC201.2
P01  (via drill 0.3)
  Top 0.406: v43.18,38.42 v43.18,67.63
  Top 0.61: IC201.4 IC201.3
  Bottom 0.406: IC101.16 v43.18,38.42 | v43.18,67.63 IC201.4
P02  (via drill 0.3)
  Top 0.406: v42.23,33.34 v42.23,62.55
  Top 0.61: IC201.5 IC201.6
  Bottom 0.406: IC101.18 v42.23,33.34 | v42.23,62.55 IC201.6
P03  (via drill 0.3)
  Top 0.406: v41.27,28.26 v41.27,57.47
  Top 0.61: IC201.8 IC201.7
  Bottom 0.406: IC101.20 v41.27,28.26 | v41.27,57.47 IC201.8
P04
  Top 0.406: IC101.29 IC202.1
  Top 0.61: IC202.2 IC202.1
P05
  Top 0.406: IC101.27 IC202.3
  Top 0.61: IC202.3 IC202.4
P06
  Top 0.406: IC101.25 IC202.5
  Top 0.61: IC202.5 IC202.6
P07
  Top 0.406: IC101.23 IC202.7
  Top 0.61: IC202.7 IC202.8
P10  (via drill 0.3)
  Top 0.406: IC101.15 20.32,40.96 16.51,44.45 16.51,51.75 16.51,55.88 v11.43,60.96
  Bottom 0.406: v11.43,60.96 11.43,69.53 9.21,71.75 X101.1
P11  (via drill 0.3)
  Top 0.406: IC101.17 21.27,35.88 12.7,44.45 12.7,57.78 v10.16,60.33
  Bottom 0.406: v10.16,60.33 10.16,67.31 9.21,68.26 6.25,68.26 X101.2
P12  (via drill 0.3)
  Top 0.406: IC101.19 22.54,30.8 8.89,44.45 v8.89,59.69
  Bottom 0.406: v8.89,59.69 8.89,63.82 7.94,64.77 5.95,64.77 X101.3
P13  (via drill 0.3)
  Top 0.406: v12.38,70.17 31.11,70.17 32.38,71.44 IC101.3
  Bottom 0.406: X101.4 3.83,61.26 2.86,62.23 2.86,73.03 3.81,73.98 8.57,73.98 v12.38,70.17
P14  (via drill 0.3)
  Top 0.406: v31.75,39.69 20,39.69 15.24,44.45 15.24,54.93 v13.97,56.2
  Bottom 0.406: IC101.28 48.58,46.04 42.23,39.69 v31.75,39.69 | v13.97,56.2 11.43,56.2 9.84,57.78 5.33,57.78 X101.5
P15  (via drill 0.3)
  Top 0.406: v31.75,37.15 21.27,37.15 13.97,44.45 v13.97,54.29
  Bottom 0.406: IC101.26 47.31,40.96 43.5,37.15 v31.75,37.15 | v13.97,54.29 5.33,54.29 X101.6
P16  (via drill 0.3)
  Top 0.406: v31.75,34.61 21.27,34.61 11.43,44.45 v11.43,50.8
  Bottom 0.406: IC101.24 36.83,35.88 35.56,34.61 v31.75,34.61 | v11.43,50.8 5.34,50.8 X101.7
P17  (via drill 0.3)
  Top 0.406: v31.75,32.07 22.54,32.07 10.16,44.45 v10.16,47.31
  Bottom 0.406: IC101.22 37.47,30.8 36.2,32.07 v31.75,32.07 | v10.16,47.31 5.35,47.31 X101.8
PLUGGED  (via drill 0.3)
  Top 0.406: v13.02,72.71 35.24,72.71 v35.56,73.03
  Bottom 0.406: IC101.39 36.51,73.98 v35.56,73.03 | CON101.3 10.65,79.84 13.02,77.47 v13.02,72.71
PWM
  Top 0.813: IC101.21 48.9,27.94 52.07,24.77 R301.2
Q-CLK  (via drill 0.3)
  Top 0.406: IC104.8 32.38,25.08 30.8,26.67 v30.8,28.26 QG101.8
  Bottom 0.406: IC101.13 30.8,43.18 v30.8,28.26
SCH-1-G  (via drill 0.3)
  Top 0.61: CON301.2 98.74,82.23 98.42,81.92 v98.42,77.79 | REL201.6 v71.12,88.9 | v79.38,88.9 v79.38,81.92
  Bottom 0.61: v98.42,77.79 94.66,77.79 X201.6 94.38,77.79 81.28,77.79 80.64,78.42 80.64,79.06 79.38,80.33 v79.38,81.92 | v71.12,88.9 v79.38,88.9
SCH-1-R
  Bottom 0.61: REL201.8 93.72,84.14 X201.4
SCH-2-G  (via drill 0.3)
  Top 0.61: CON302.2 98.74,57.78 98.42,57.47 v98.42,53.34 | v74.61,50.8 74.61,62.87 74.93,63.18 REL202.6
  Bottom 0.61: v98.42,53.34 94.66,53.34 X202.6 92.53,53.48 90.81,51.75 88.9,51.75 87.95,50.8 v74.61,50.8
SCH-2-R  (via drill 0.3)
  Top 0.813: v87.95,62.55 v87.95,60.33
  Bottom 0.813: REL202.8 81.92,62.55 v87.95,62.55 | v87.95,60.33 94.36,60.33 X202.4
SCH-3-G  (via drill 0.3)
  Top 0.61: CON303.2 98.74,33.34 98.42,33.02 v98.42,28.89 | v77.79,33.66 77.79,37.78 REL203.6
  Bottom 0.61: v98.42,28.89 94.66,28.89 X203.6 94.52,28.71 85.9,28.71 80.96,33.66 v77.79,33.66
SCH-3-R  (via drill 0.3)
  Top 0.813: v87.95,39.05 v87.95,35.88
  Bottom 0.813: REL203.8 81.6,39.05 v87.95,39.05 | v87.95,35.88 94.36,35.88 X203.4
SCH-4-G  (via drill 0.3)
  Top 0.61: CON304.2 98.74,8.89 98.42,8.57 v98.42,4.45 | v84.45,4.76 v84.45,7.94 | v79.06,7.94 v79.06,18.41
  Bottom 0.61: v98.42,4.45 94.66,4.45 X204.6 84.63,4.58 v84.45,4.76 | v84.45,7.94 v79.06,7.94 | v79.06,18.41 REL204.6
SCH-4-R  (via drill 0.3)
  Top 0.61: REL204.8 v81.28,11.43
  Bottom 0.61: v81.28,11.43 94.36,11.43 X204.4
SCK  (via drill 0.3)
  Top 0.406: v36.51,58.74 36.51,26.04 36.2,25.72 36.2,20 v37.47,18.41 IC104.13 37.47,14.92 36.2,13.65 36.2,3.49 36.83,2.86 44.45,2.86 45.09,3.49 IC102.6
  Bottom 0.406: IC101.8 v36.51,58.74 | SV101.3 20.95,13.97 20,14.92 20,17.46 20.95,18.41 v37.47,18.41
SEL1  (via drill 0.3)
  Top 0.61: LED205.K 89.53,81.6 89.53,91.76 LED206.A v87.95,96.84 | REL201.13 65.41,91.76 64.77,92.39 64.77,98.42 65.41,99.06 81.28,99.06 v83.5,96.84 | v54.61,66.36 v54.61,77.79 | v73.98,80.01 73.98,89.22 73.34,89.85 70.8,89.85 v69.85,88.9
  Bottom 0.61: v83.5,96.84 v87.95,96.84 | IC101.36 v54.61,66.36 | v54.61,77.79 59.37,77.79 60.33,78.74 72.71,78.74 v73.98,80.01 | v69.85,88.9 65.09,88.9 64.77,89.22 64.77,90.49 REL201.13
SEL2  (via drill 0.3)
  Top 0.61: LED201.K 89.53,57.15 89.53,67.31 LED202.A | v71.12,67.31 REL202.13
  Bottom 0.61: LED202.A 87.31,68.9 85.72,67.31 v71.12,67.31 63.82,67.31 62.87,66.36 57.78,66.36 55.24,63.82 IC101.35
SEL3  (via drill 0.3)
  Top 0.61: LED207.K 89.53,32.7 89.53,42.86 LED208.A v87.95,49.85 | REL203.13 v71.12,49.85
  Bottom 0.61: v87.95,49.85 v71.12,49.85 69.22,49.85 67.94,51.12 62.55,51.12 61.91,51.75 61.91,52.39 60.96,53.34 57.47,53.34 56.83,53.98 56.83,60.01 55.56,61.28 IC101.34
SEL4  (via drill 0.3)
  Top 0.61: LED203.K 89.53,8.26 89.53,18.41 LED204.A v87.95,27.62 | v74.61,26.04 v74.61,32.7 | v46.99,32.07 46.99,58.42 47.31,58.74 IC101.33
  Bottom 0.61: REL204.13 v74.61,26.04 | v87.95,27.62 85.41,27.62 80.33,32.7 v74.61,32.7 63.18,32.7 62.55,32.07 v46.99,32.07
SPG
  Top 0.406: R107.2 R108.1 45.72,77.15 46.35,76.52 IC101.40
V-NETZTEIL1
  Top 1.016: CON101.1 19.05,90.49 21.91,93.34 D103.A

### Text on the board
Bottom: MBCAN-Projekt | (c) Dr.-Ing. Th. Wiesner | 23.03.2024 | mbc83.brd | bottom
tNames: HW: 24.03.23 | +18V | DC | (c) Dr.-Ing. Th. Wiesner | MBCAN-Projekt | IN | OUT | mbc-83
